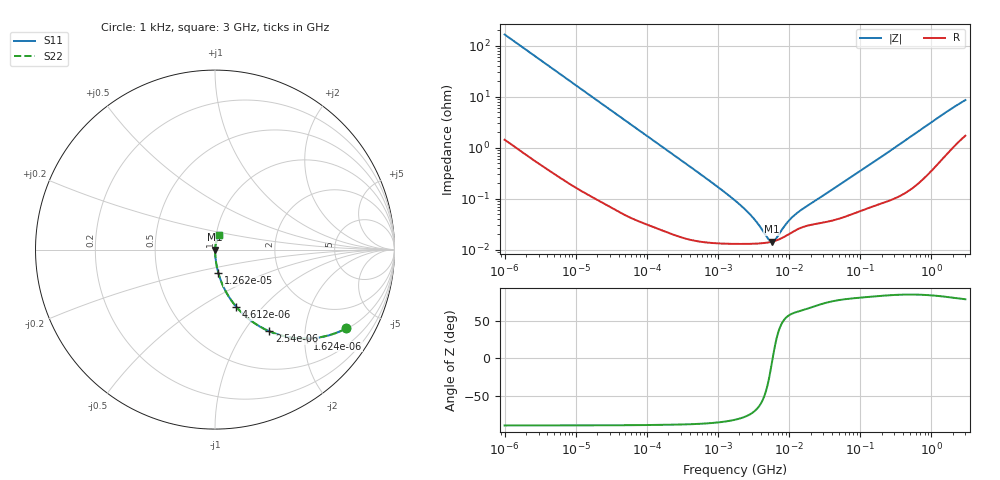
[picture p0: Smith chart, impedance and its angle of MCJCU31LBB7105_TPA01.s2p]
! MCJCU31LBB7105_TPA01  S-PARAMETER MODEL  ( Standard Model )
! Model Generated by TAIYO YUDEN Corporation (http://www.ty-top.com)
! Version 1.0
! TAIYO YUDEN Control No. 220601
! Copyright(c) 2015 TAIYO YUDEN CO.,LTD. All Rights Reserved.
! Product Description (link to TY-COMPAS)
! https://ds.yuden.co.jp/TYCOMPAS/or/detail?pn=MCJCU31LBB7105KTPA01&u=M
! Products Name : Multilayer Ceramic Capacitors
! Characteristics :
!  Capacitance : 1 [uF] , Rated Voltage : 50 [V] , TCC : X7R
!  Case Size : 3.2 x 1.6 / 0.126 x 0.063 [mm/inch] , Thickness : 1.6 / 0.063 [mm/inch]
!  (Conditions: Temperature = 25 [degC] , DC Bias Voltage = 0 [V])
! External Node Assignments :
!  1  o---| |---o  2
! GND o---------o GND
! Frequency Range : 1kHz  -  3GHz  [ 401 STEP ]
# MHZ S RI R 50
! Freq[MHz].  S11 Real  S11 Imag  S21 Real  S21 Imag  S12 Real  S12 Imag  S22 Real  S22 Imag
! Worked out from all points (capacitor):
!   401 points, 1 kHz to 3 GHz, reference 50 ohm
!   read as one part in series: C = 956 nF near 1.077 kHz
!   lowest |Z| = 14.4 mohm at 5.711 MHz (marker M1)
!   series resonance near 5.864 MHz, so ESL is about 770 pH
!   S11 on the Smith chart (normalised r, x): 1 kHz: 1.03, -3.32; 1.624 kHz: 1.02, -2.05; 2.54 kHz: 1.01, -1.31; 4.612 kHz: 1.01, -0.73; 12.62 kHz: 1.00, -0.27; 3 GHz: 1.03, +0.17
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0.001  0.7322 -0.4385  0.2678 0.4385  0.2678 0.4385  0.7322 -0.4385
0.001624  0.5127 -0.4955  0.4873 0.4955  0.4873 0.4955  0.5127 -0.4955
0.00254  0.3034 -0.4554  0.6966 0.4554  0.6966 0.4554  0.3034 -0.4554
0.004612  0.1188 -0.319  0.8812 0.319  0.8812 0.319  0.1188 -0.319
0.006951  0.057 -0.2273  0.943 0.2273  0.943 0.2273  0.057 -0.2273
0.01216  0.0201 -0.1355  0.9799 0.1355  0.9799 0.1355  0.0201 -0.1355
0.012621  0.0188 -0.1308  0.9812 0.1308  0.9812 0.1308  0.0188 -0.1308
0.03454  0.00302 -0.0489  0.997 0.0489  0.997 0.0489  0.00302 -0.0489
0.147855  0.000386 -0.0116  0.9996 0.0116  0.9996 0.0116  0.000386 -0.0116
0.762639  0.000141 -0.00223  0.9999 0.00223  0.9999 0.00223  0.000141 -0.00223
1.732051  0.000131 -0.000914  0.9999 0.000914  0.9999 0.000914  0.000131 -0.000914
2.919173  0.000131 -0.000449  0.9999 0.000449  0.9999 0.000449  0.000131 -0.000449
3.651041  0.000132 -0.000293  0.9999 0.000293  0.9999 0.000293  0.000132 -0.000293
5.106836  0.000139 -8.27e-05  0.9999 8.27e-05  0.9999 8.27e-05  0.000139 -8.27e-05
5.711239  0.000143 -1.56e-05  0.9999 1.56e-05  0.9999 1.56e-05  0.000143 -1.56e-05
6.387174  0.00015 5.11e-05  0.9999 -5.11e-05  0.9999 -5.11e-05  0.00015 5.11e-05
8.933959  0.000185 0.000251  0.9998 -0.000251  0.9998 -0.000251  0.000185 0.000251
11.1738  0.000223 0.00038  0.9998 -0.00038  0.9998 -0.00038  0.000223 0.00038
21.06097  0.000311 0.000772  0.9997 -0.000772  0.9997 -0.000772  0.000311 0.000772
256.0921  0.000985 0.00841  0.999 -0.00841  0.999 -0.00841  0.000985 0.00841
1371.11  0.00739 0.0421  0.9926 -0.0421  0.9926 -0.0421  0.00739 0.0421
3000  0.0236 0.0809  0.9764 -0.0809  0.9764 -0.0809  0.0236 0.0809
